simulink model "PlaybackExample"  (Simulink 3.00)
settings: Solver=FixedStepDiscrete  StartTime=0.0  StopTime=20.0  FixedStep=0.05  RelTol=1e-3
libraries: AVDSBlockset x11, simulink3 x1

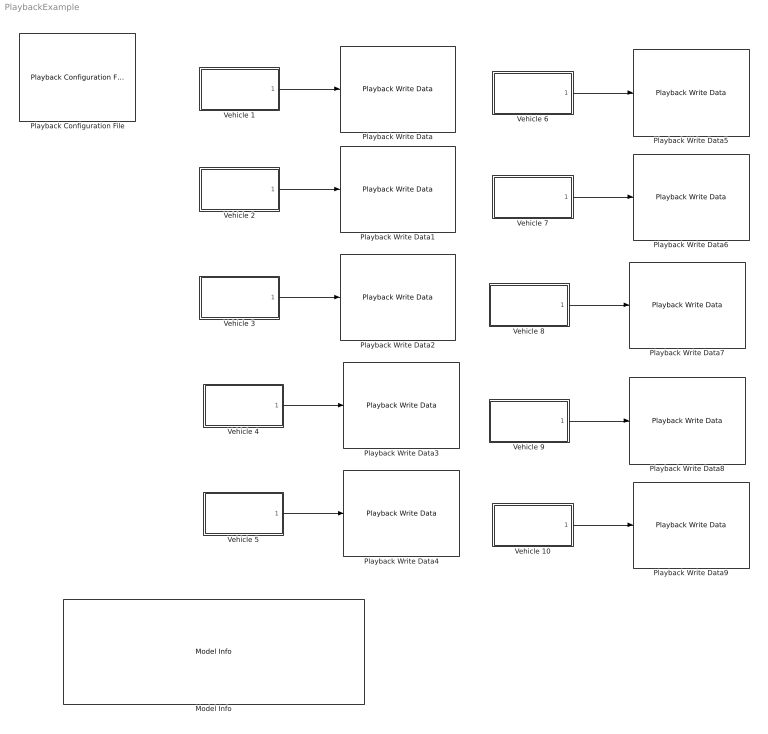
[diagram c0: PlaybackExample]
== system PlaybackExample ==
  Model Info : simulink3/Signals & Systems/Model Info  InitialBlockCM=none  BlockCM=none  Frame=off  DisplayStringWithTags=|  HorizontalTextAlignment=Left  LeftAlignmentValue=0.02  SourceBlockDiagram=PlaybackExample  TagMaxNumber=20
      | PlaybackExample.mdl - Simulink example that saves multiple vehicle trajectories into
      |    data files for AVDS plaback.
      |    - Open the PlaybackExample model file.
      |    - Run the Simulink simulation.
      |    - Run AVDS
      |    - In AVDS, load the file, 'SimulinkExample.ply.ini', to do this from AVDS's 
      |      menu select "File->Playback Init->Open". Note, this file will be located in the 
      |      directory "AVDS\Utilit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
  Playback Configuration File : AVDSBlockset/Playback Configuration File  ConfigurationFileName=SimulinkConfiguration.ply.ini  DataFileNameBase=SimulinkData  NumberVehicles=10
  Playback Write Data : AVDSBlockset/Playback Write Data  DataFileNameBase=SimulinkData  VehicleID=01  NumberDataSignals=7
  Playback Write Data1 : AVDSBlockset/Playback Write Data  DataFileNameBase=SimulinkData  VehicleID=02  NumberDataSignals=7
  Playback Write Data2 : AVDSBlockset/Playback Write Data  DataFileNameBase=SimulinkData  VehicleID=03  NumberDataSignals=7
  Playback Write Data3 : AVDSBlockset/Playback Write Data  DataFileNameBase=SimulinkData  VehicleID=04  NumberDataSignals=7
  Playback Write Data4 : AVDSBlockset/Playback Write Data  DataFileNameBase=SimulinkData  VehicleID=05  NumberDataSignals=7
  Playback Write Data5 : AVDSBlockset/Playback Write Data  DataFileNameBase=SimulinkData  VehicleID=06  NumberDataSignals=7
  Playback Write Data6 : AVDSBlockset/Playback Write Data  DataFileNameBase=SimulinkData  VehicleID=07  NumberDataSignals=7
  Playback Write Data7 : AVDSBlockset/Playback Write Data  DataFileNameBase=SimulinkData  VehicleID=08  NumberDataSignals=7
  Playback Write Data8 : AVDSBlockset/Playback Write Data  DataFileNameBase=SimulinkData  VehicleID=09  NumberDataSignals=7
  Playback Write Data9 : AVDSBlockset/Playback Write Data  DataFileNameBase=SimulinkData  VehicleID=10  NumberDataSignals=7
  Vehicle 1 : Subsystem
  Vehicle 10 : Subsystem
  Vehicle 2 : Subsystem
  Vehicle 3 : Subsystem
  Vehicle 4 : Subsystem
  Vehicle 5 : Subsystem
  Vehicle 6 : Subsystem
  Vehicle 7 : Subsystem
  Vehicle 8 : Subsystem
  Vehicle 9 : Subsystem
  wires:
  Vehicle 1/1(Vehicle Output) -> Playback Write Data/1
  Vehicle 2/1(Vehicle Output) -> Playback Write Data1/1
  Vehicle 3/1(Vehicle Output) -> Playback Write Data2/1
  Vehicle 4/1(Vehicle Output) -> Playback Write Data3/1
  Vehicle 5/1(Vehicle Output) -> Playback Write Data4/1
  Vehicle 6/1(Vehicle Output) -> Playback Write Data5/1
  Vehicle 7/1(Vehicle Output) -> Playback Write Data6/1
  Vehicle 8/1(Vehicle Output) -> Playback Write Data7/1
  Vehicle 9/1(Vehicle Output) -> Playback Write Data8/1
  Vehicle 10/1(Vehicle Output) -> Playback Write Data9/1

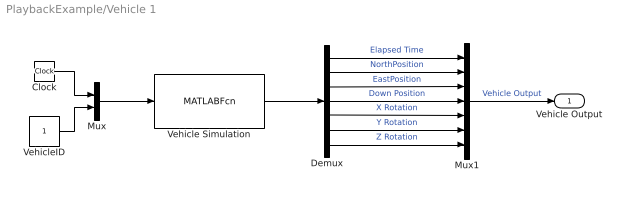
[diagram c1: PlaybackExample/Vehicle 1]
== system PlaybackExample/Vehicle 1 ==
  Clock : Clock
  Demux : Demux  Outputs=7
  Mux : Mux  Inputs=2
  Mux1 : Mux  Inputs=7
  Vehicle Simulation : MATLABFcn  MATLABFcn=SimulinkVehicle  OutputWidth=7  OutputSignalType=auto
  VehicleID : Constant  Value=1
  Vehicle Output : Outport  Port=1
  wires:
  Vehicle Simulation/1 -> Demux/1
  Mux1/1 -> Vehicle Output/1  "Vehicle Output"
  Demux/1 -> Mux1/1  "Elapsed Time"
  Demux/2 -> Mux1/2  "NorthPosition"
  Demux/3 -> Mux1/3  "EastPosition"
  Demux/4 -> Mux1/4  "Down Position"
  Demux/5 -> Mux1/5  "X Rotation"
  Demux/6 -> Mux1/6  "Y Rotation"
  Demux/7 -> Mux1/7  "Z Rotation"
  Mux/1 -> Vehicle Simulation/1
  Clock/1 -> Mux/1
  VehicleID/1 -> Mux/2

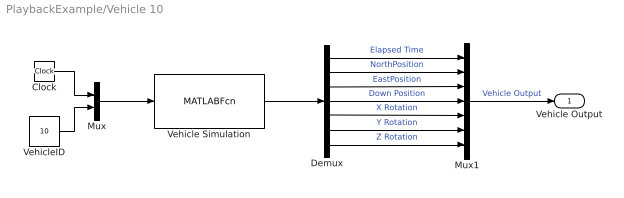
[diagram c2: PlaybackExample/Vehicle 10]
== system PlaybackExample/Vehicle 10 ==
  Clock : Clock
  Demux : Demux  Outputs=7
  Mux : Mux  Inputs=2
  Mux1 : Mux  Inputs=7
  Vehicle Simulation : MATLABFcn  MATLABFcn=SimulinkVehicle  OutputWidth=7  OutputSignalType=auto
  VehicleID : Constant  Value=10
  Vehicle Output : Outport  Port=1
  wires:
  VehicleID/1 -> Mux/2
  Clock/1 -> Mux/1
  Mux/1 -> Vehicle Simulation/1
  Demux/7 -> Mux1/7  "Z Rotation"
  Demux/6 -> Mux1/6  "Y Rotation"
  Demux/5 -> Mux1/5  "X Rotation"
  Demux/4 -> Mux1/4  "Down Position"
  Demux/3 -> Mux1/3  "EastPosition"
  Demux/2 -> Mux1/2  "NorthPosition"
  Demux/1 -> Mux1/1  "Elapsed Time"
  Mux1/1 -> Vehicle Output/1  "Vehicle Output"
  Vehicle Simulation/1 -> Demux/1

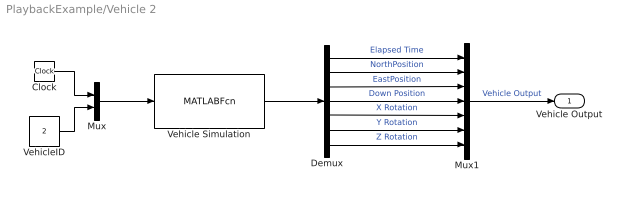
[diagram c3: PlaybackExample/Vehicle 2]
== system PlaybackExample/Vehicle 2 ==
  Clock : Clock
  Demux : Demux  Outputs=7
  Mux : Mux  Inputs=2
  Mux1 : Mux  Inputs=7
  Vehicle Simulation : MATLABFcn  MATLABFcn=SimulinkVehicle  OutputWidth=7  OutputSignalType=auto
  VehicleID : Constant  Value=2
  Vehicle Output : Outport  Port=1
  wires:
  VehicleID/1 -> Mux/2
  Clock/1 -> Mux/1
  Mux/1 -> Vehicle Simulation/1
  Demux/7 -> Mux1/7  "Z Rotation"
  Demux/6 -> Mux1/6  "Y Rotation"
  Demux/5 -> Mux1/5  "X Rotation"
  Demux/4 -> Mux1/4  "Down Position"
  Demux/3 -> Mux1/3  "EastPosition"
  Demux/2 -> Mux1/2  "NorthPosition"
  Demux/1 -> Mux1/1  "Elapsed Time"
  Mux1/1 -> Vehicle Output/1  "Vehicle Output"
  Vehicle Simulation/1 -> Demux/1

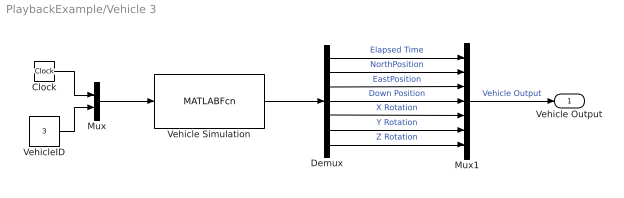
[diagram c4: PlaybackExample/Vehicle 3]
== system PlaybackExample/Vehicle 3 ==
  Clock : Clock
  Demux : Demux  Outputs=7
  Mux : Mux  Inputs=2
  Mux1 : Mux  Inputs=7
  Vehicle Simulation : MATLABFcn  MATLABFcn=SimulinkVehicle  OutputWidth=7  OutputSignalType=auto
  VehicleID : Constant  Value=3
  Vehicle Output : Outport  Port=1
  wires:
  Vehicle Simulation/1 -> Demux/1
  Mux1/1 -> Vehicle Output/1  "Vehicle Output"
  Demux/1 -> Mux1/1  "Elapsed Time"
  Demux/2 -> Mux1/2  "NorthPosition"
  Demux/3 -> Mux1/3  "EastPosition"
  Demux/4 -> Mux1/4  "Down Position"
  Demux/5 -> Mux1/5  "X Rotation"
  Demux/6 -> Mux1/6  "Y Rotation"
  Demux/7 -> Mux1/7  "Z Rotation"
  Mux/1 -> Vehicle Simulation/1
  Clock/1 -> Mux/1
  VehicleID/1 -> Mux/2

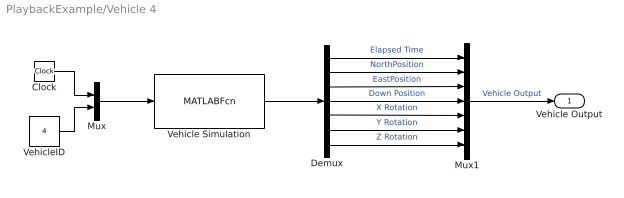
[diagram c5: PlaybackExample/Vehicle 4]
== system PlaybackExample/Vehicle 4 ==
  Clock : Clock
  Demux : Demux  Outputs=7
  Mux : Mux  Inputs=2
  Mux1 : Mux  Inputs=7
  Vehicle Simulation : MATLABFcn  MATLABFcn=SimulinkVehicle  OutputWidth=7  OutputSignalType=auto
  VehicleID : Constant  Value=4
  Vehicle Output : Outport  Port=1
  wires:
  VehicleID/1 -> Mux/2
  Clock/1 -> Mux/1
  Mux/1 -> Vehicle Simulation/1
  Demux/7 -> Mux1/7  "Z Rotation"
  Demux/6 -> Mux1/6  "Y Rotation"
  Demux/5 -> Mux1/5  "X Rotation"
  Demux/4 -> Mux1/4  "Down Position"
  Demux/3 -> Mux1/3  "EastPosition"
  Demux/2 -> Mux1/2  "NorthPosition"
  Demux/1 -> Mux1/1  "Elapsed Time"
  Mux1/1 -> Vehicle Output/1  "Vehicle Output"
  Vehicle Simulation/1 -> Demux/1

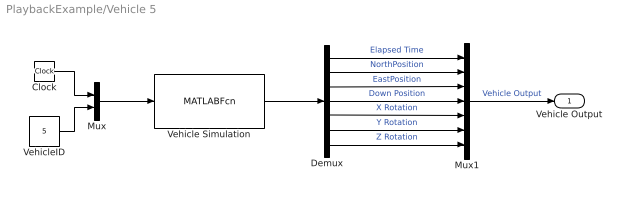
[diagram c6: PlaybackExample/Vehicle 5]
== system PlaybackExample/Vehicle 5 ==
  Clock : Clock
  Demux : Demux  Outputs=7
  Mux : Mux  Inputs=2
  Mux1 : Mux  Inputs=7
  Vehicle Simulation : MATLABFcn  MATLABFcn=SimulinkVehicle  OutputWidth=7  OutputSignalType=auto
  VehicleID : Constant  Value=5
  Vehicle Output : Outport  Port=1
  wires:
  Vehicle Simulation/1 -> Demux/1
  Mux1/1 -> Vehicle Output/1  "Vehicle Output"
  Demux/1 -> Mux1/1  "Elapsed Time"
  Demux/2 -> Mux1/2  "NorthPosition"
  Demux/3 -> Mux1/3  "EastPosition"
  Demux/4 -> Mux1/4  "Down Position"
  Demux/5 -> Mux1/5  "X Rotation"
  Demux/6 -> Mux1/6  "Y Rotation"
  Demux/7 -> Mux1/7  "Z Rotation"
  Mux/1 -> Vehicle Simulation/1
  Clock/1 -> Mux/1
  VehicleID/1 -> Mux/2

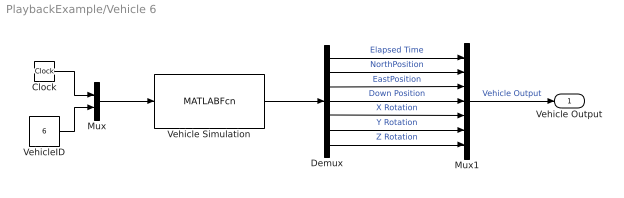
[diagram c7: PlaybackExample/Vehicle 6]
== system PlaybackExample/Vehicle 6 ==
  Clock : Clock
  Demux : Demux  Outputs=7
  Mux : Mux  Inputs=2
  Mux1 : Mux  Inputs=7
  Vehicle Simulation : MATLABFcn  MATLABFcn=SimulinkVehicle  OutputWidth=7  OutputSignalType=auto
  VehicleID : Constant  Value=6
  Vehicle Output : Outport  Port=1
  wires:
  VehicleID/1 -> Mux/2
  Clock/1 -> Mux/1
  Mux/1 -> Vehicle Simulation/1
  Demux/7 -> Mux1/7  "Z Rotation"
  Demux/6 -> Mux1/6  "Y Rotation"
  Demux/5 -> Mux1/5  "X Rotation"
  Demux/4 -> Mux1/4  "Down Position"
  Demux/3 -> Mux1/3  "EastPosition"
  Demux/2 -> Mux1/2  "NorthPosition"
  Demux/1 -> Mux1/1  "Elapsed Time"
  Mux1/1 -> Vehicle Output/1  "Vehicle Output"
  Vehicle Simulation/1 -> Demux/1

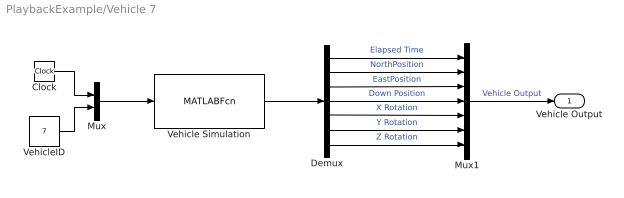
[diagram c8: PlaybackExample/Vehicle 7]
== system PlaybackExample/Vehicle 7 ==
  Clock : Clock
  Demux : Demux  Outputs=7
  Mux : Mux  Inputs=2
  Mux1 : Mux  Inputs=7
  Vehicle Simulation : MATLABFcn  MATLABFcn=SimulinkVehicle  OutputWidth=7  OutputSignalType=auto
  VehicleID : Constant  Value=7
  Vehicle Output : Outport  Port=1
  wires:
  Vehicle Simulation/1 -> Demux/1
  Mux1/1 -> Vehicle Output/1  "Vehicle Output"
  Demux/1 -> Mux1/1  "Elapsed Time"
  Demux/2 -> Mux1/2  "NorthPosition"
  Demux/3 -> Mux1/3  "EastPosition"
  Demux/4 -> Mux1/4  "Down Position"
  Demux/5 -> Mux1/5  "X Rotation"
  Demux/6 -> Mux1/6  "Y Rotation"
  Demux/7 -> Mux1/7  "Z Rotation"
  Mux/1 -> Vehicle Simulation/1
  Clock/1 -> Mux/1
  VehicleID/1 -> Mux/2

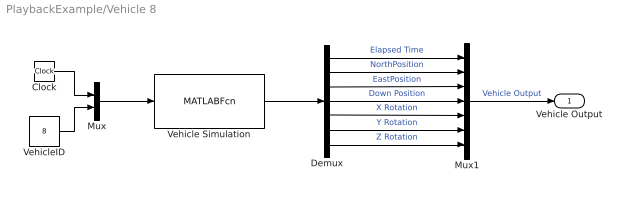
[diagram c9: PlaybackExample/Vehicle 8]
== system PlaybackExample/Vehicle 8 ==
  Clock : Clock
  Demux : Demux  Outputs=7
  Mux : Mux  Inputs=2
  Mux1 : Mux  Inputs=7
  Vehicle Simulation : MATLABFcn  MATLABFcn=SimulinkVehicle  OutputWidth=7  OutputSignalType=auto
  VehicleID : Constant  Value=8
  Vehicle Output : Outport  Port=1
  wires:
  VehicleID/1 -> Mux/2
  Clock/1 -> Mux/1
  Mux/1 -> Vehicle Simulation/1
  Demux/7 -> Mux1/7  "Z Rotation"
  Demux/6 -> Mux1/6  "Y Rotation"
  Demux/5 -> Mux1/5  "X Rotation"
  Demux/4 -> Mux1/4  "Down Position"
  Demux/3 -> Mux1/3  "EastPosition"
  Demux/2 -> Mux1/2  "NorthPosition"
  Demux/1 -> Mux1/1  "Elapsed Time"
  Mux1/1 -> Vehicle Output/1  "Vehicle Output"
  Vehicle Simulation/1 -> Demux/1

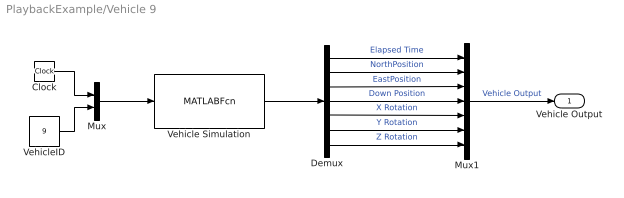
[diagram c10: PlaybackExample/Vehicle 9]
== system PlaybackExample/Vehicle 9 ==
  Clock : Clock
  Demux : Demux  Outputs=7
  Mux : Mux  Inputs=2
  Mux1 : Mux  Inputs=7
  Vehicle Simulation : MATLABFcn  MATLABFcn=SimulinkVehicle  OutputWidth=7  OutputSignalType=auto
  VehicleID : Constant  Value=9
  Vehicle Output : Outport  Port=1
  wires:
  Vehicle Simulation/1 -> Demux/1
  Mux1/1 -> Vehicle Output/1  "Vehicle Output"
  Demux/1 -> Mux1/1  "Elapsed Time"
  Demux/2 -> Mux1/2  "NorthPosition"
  Demux/3 -> Mux1/3  "EastPosition"
  Demux/4 -> Mux1/4  "Down Position"
  Demux/5 -> Mux1/5  "X Rotation"
  Demux/6 -> Mux1/6  "Y Rotation"
  Demux/7 -> Mux1/7  "Z Rotation"
  Mux/1 -> Vehicle Simulation/1
  Clock/1 -> Mux/1
  VehicleID/1 -> Mux/2
